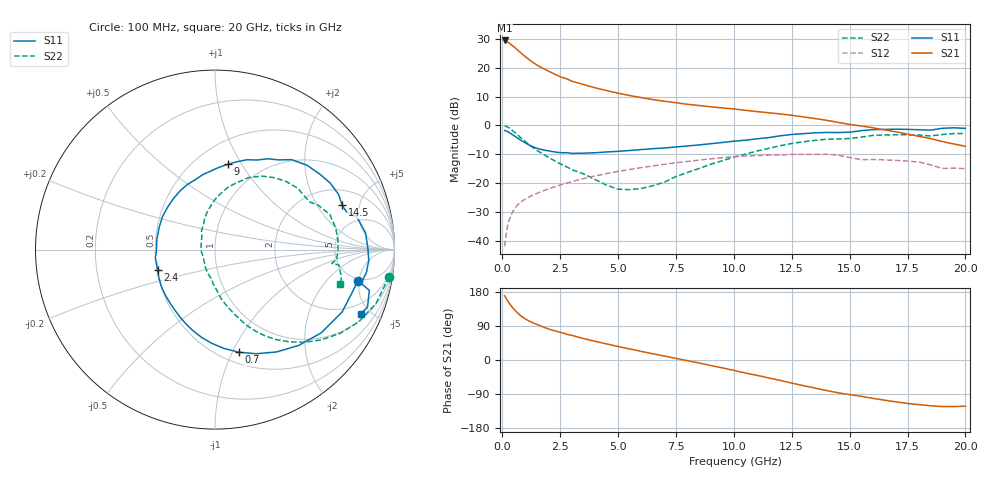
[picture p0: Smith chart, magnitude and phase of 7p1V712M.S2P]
! Infineon Technologies  Discrete & RF Semiconductors
! bfp620
! VCE =  1.7 V,  IC =  12 mA
! Common Emitter S-Parameters:  Sep 2002
# GHz  S  MA  R  50
!  f  S11  S21  S12  S22
! GHz  MAG  ANG  MAG  ANG  MAG  ANG  MAG  ANG
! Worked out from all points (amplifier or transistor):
!   59 points, 100 MHz to 20 GHz, reference 50 ohm
!   highest |S21| = 29.5 dB at 100 MHz (marker M1)
!   |S21| within 3 dB of that: start of sweep to 614.2 MHz
!   unconditionally stable (mu >= 1): 3.905 GHz to 10.43 GHz; 17.11 GHz to end of sweep
!   at 1 GHz: K = 0.54, MSG = 24.7 dB, |S12| = -25.5 dB
!   at 5.5 GHz: K = 1.04, MAG = 11.6 dB, |S12| = -15.3 dB
!   at 20 GHz: K = 1.33, MAG = 0.4 dB, |S12| = -15.0 dB
!   S11 on the Smith chart (normalised r, x): 100 MHz: 4.73, -4.88; 700 MHz: 0.61, -1.06; 2.4 GHz: 0.50, -0.13; 9 GHz: 0.71, +0.87; 14.5 GHz: 3.00, +3.38; 20 GHz: 1.31, -4.40
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0.1  0.8162 -12.2  29.8 169.4  0.008 76.8  0.9809 -8.9
0.2  0.7891 -26.1  28.49 158.9  0.016 75.8  0.9461 -18.6
0.3  0.7517 -38.1  26.82 149.8  0.0229 71.6  0.8962 -26.7
0.4  0.7088 -48.9  24.99 141.7  0.0289 67.4  0.838 -33.9
0.5  0.6653 -59.0  23.13 134.4  0.0342 63.7  0.7771 -40.3
0.6  0.6241 -68.4  21.34 127.9  0.0389 60.5  0.7176 -46.0
0.7  0.5865 -77.0  19.68 122.0  0.043 57.9  0.6615 -51.0
0.8  0.5525 -84.9  18.16 116.8  0.0467 55.8  0.6098 -55.5
1  0.4942 -98.8  15.54 108.2  0.0529 52.7  0.5207 -62.6
1.3  0.4288 -115.8  12.57 98.9  0.0609 49.9  0.4189 -69.9
1.8  0.373 -138.6  9.562 86.3  0.0739 47.1  0.3097 -79.2
2.4  0.3393 -160.5  7.287 74.9  0.0895 44.1  0.2262 -87.5
3  0.3265 -178.6  5.858 65.1  0.1054 40.4  0.1704 -95.2
3.5  0.3292 169.5  5.131 56.6  0.1192 37.1  0.1446 -104.0
5  0.3544 138.2  3.623 35.6  0.1589 25.6  0.0781 -146.5
7  0.4047 105.8  2.62 10.6  0.2111 8.4  0.1033 135.1
9  0.4805 81.5  2.104 -14.4  0.2624 -11.4  0.2113 102.3
10.5  0.5528 64.6  1.825 -34.3  0.294 -29.0  0.3169 83.8
13.5  0.7411 30.1  1.315 -74.0  0.3144 -63.3  0.549 43.8
14.5  0.7502 19.2  1.127 -86.5  0.3038 -78.2  0.5809 30.7
17  0.8589 -4.0  0.773 -110.5  0.2464 -94.5  0.6868 4.8
20  0.8876 -23.7  0.433 -122.1  0.1772 -105.7  0.7242 -15.2
